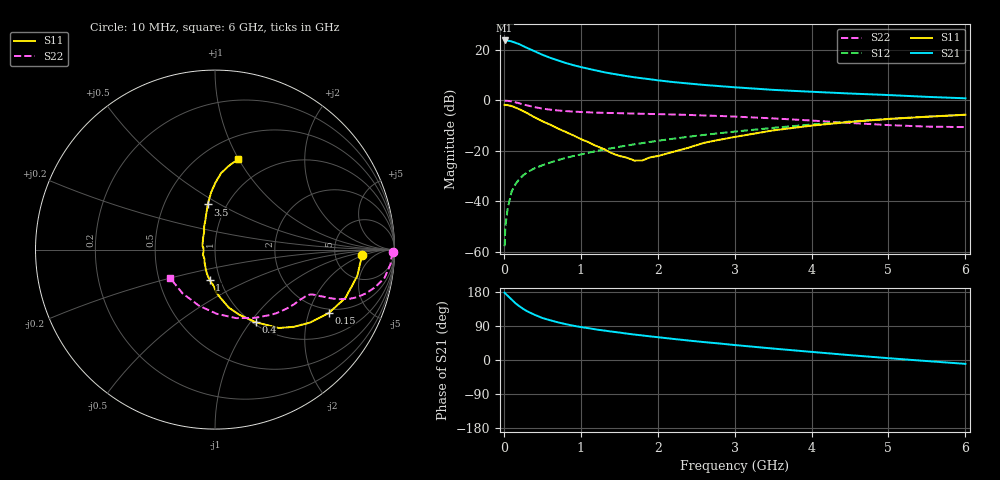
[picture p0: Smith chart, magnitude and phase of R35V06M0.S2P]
! SIEMENS Small Signal Semiconductors
! BFR181
! Si NPN RF Bipolar Junction Transistor in SOT23
! VCE = 5 V  IC = 6 mA
! Common Emitter S-Parameters:  May  1996
# GHz  S  MA  R  50
!  f  S11  S21  S12  S22
! GHz  MAG  ANG  MAG  ANG  MAG  ANG  MAG  ANG
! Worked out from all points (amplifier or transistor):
!   36 points, 10 MHz to 6 GHz, reference 50 ohm
!   highest |S21| = 23.8 dB at 10 MHz (marker M1)
!   |S21| within 3 dB of that: start of sweep to 305.4 MHz
!   unconditionally stable (mu >= 1): 1.061 GHz to 2.917 GHz
!   at 250 MHz: K = 0.46, MSG = 25.6 dB, |S12| = -29.7 dB
!   at 1.4 GHz: K = 1.05, MAG = 13.5 dB, |S12| = -18.9 dB
!   at 6 GHz: K = 0.86, MSG = 3.3 dB, |S12| = -5.7 dB
!   S11 on the Smith chart (normalised r, x): 10 MHz: 9.63, -1.83; 150 MHz: 1.82, -2.72; 400 MHz: 1.03, -1.06; 1 GHz: 0.89, -0.31; 3.5 GHz: 0.82, +0.44; 6 GHz: 0.72, +1.00
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0.01  0.8179 -2.2  15.41 177.5  0.0013 94.0  0.9903 -0.9
0.02  0.8156 -3.9  15.2 175.4  0.0032 87.6  0.9859 -1.9
0.05  0.8064 -10.5  15.31 169.5  0.0072 84.7  0.9811 -4.8
0.1  0.7751 -20.3  14.79 159.9  0.0155 80.2  0.9579 -9.4
0.15  0.7252 -29.2  13.89 149.9  0.0219 75.3  0.9183 -13.1
0.2  0.6686 -37.4  13.03 142.1  0.0275 72.2  0.8768 -16.1
0.25  0.6156 -44.3  11.97 135.1  0.0327 68.9  0.8356 -18.5
0.3  0.563 -50.9  11 128.9  0.0375 67.8  0.8001 -20.0
0.4  0.4642 -60.7  9.417 119.3  0.0454 65.8  0.7383 -22.0
0.5  0.3878 -69.5  8.033 110.9  0.0519 65.3  0.6898 -23.0
0.6  0.3322 -76.6  7.021 105.0  0.0587 65.0  0.6579 -23.5
0.7  0.2796 -82.3  6.223 99.6  0.0656 65.1  0.6343 -24.0
0.8  0.2391 -88.3  5.544 94.8  0.0723 64.8  0.6168 -24.3
1  0.1719 -100.0  4.593 87.0  0.085 65.8  0.5908 -25.0
1.1  0.149 -106.4  4.237 83.9  0.0921 66.1  0.5817 -25.6
1.3  0.1091 -119.5  3.631 77.8  0.1067 66.1  0.5684 -27.1
1.6  0.0732 -155.9  3.026 69.6  0.1279 65.5  0.5543 -29.8
2.2  0.0958 133.3  2.312 55.7  0.1745 63.4  0.527 -36.9
3.5  0.2551 99.1  1.62 30.2  0.2866 54.1  0.4409 -59.6
4.5  0.3753 89.5  1.371 12.8  0.383 43.7  0.358 -88.4
5.5  0.476 80.3  1.178 -2.8  0.4767 31.3  0.3034 -126.7
6  0.5215 75.5  1.102 -10.2  0.5201 24.3  0.2962 -148.2
